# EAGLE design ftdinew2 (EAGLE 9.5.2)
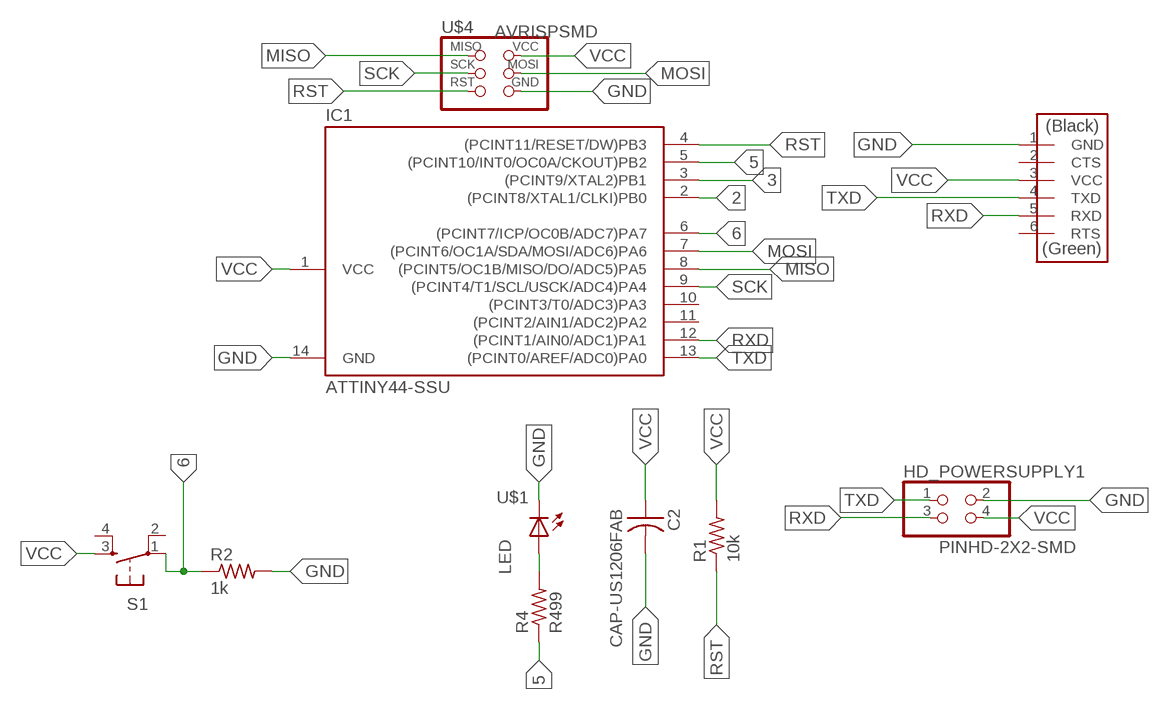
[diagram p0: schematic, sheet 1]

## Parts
C2  CAP-US1206FAB  [C1206FAB]
HD_POWERSUPPLY1  PINHD-2X2-SMD  [2X02SMD]
IC1  ATTINY44-SSU  [SOIC14]
R1  10k  RES-US1206  [R1206]
R2  1k  RES-US1206  [R1206]
R4  R499  RES-US1206  [R1206]
S1  6MM_SWITCH6MM_SWITCH  [6MM_SWITCH]
U$1  LED  [LED1206]
U$4  AVRISPSMD  [2X03SMD]
U$5  FTDI-SMD-HEADER  [1X06SMD]

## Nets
2: IC1.2((PCINT8/XTAL1/CLKI)PB0)
3: IC1.3((PCINT9/XTAL2)PB1)
5: IC1.5((PCINT10/INT0/OC0A/CKOUT)PB2) R4.1
6: IC1.6((PCINT7/ICP/OC0B/ADC7)PA7) R2.1 S1.1(P)
GND: C2.2 HD_POWERSUPPLY1.2 IC1.14(GND) R2.2 U$1.2(C) U$4.6(GND) U$5.1(GND)
MISO: IC1.8((PCINT5/OC1B/MISO/DO/ADC5)PA5) U$4.1(MISO)
MOSI: IC1.7((PCINT6/OC1A/SDA/MOSI/ADC6)PA6) U$4.4(MOSI)
N$1: R4.2 U$1.1(A)
RST: IC1.4((PCINT11/RESET/DW)PB3) R1.1 U$4.5(RST)
RXD: HD_POWERSUPPLY1.3 IC1.12((PCINT1/AIN0/ADC1)PA1) U$5.5(RXD)
SCK: IC1.9((PCINT4/T1/SCL/USCK/ADC4)PA4) U$4.3(SCK)
TXD: HD_POWERSUPPLY1.1 IC1.13((PCINT0/AREF/ADC0)PA0) U$5.4(TXD)
VCC: C2.1 HD_POWERSUPPLY1.4 IC1.1(VCC) R1.2 S1.3(S) U$4.2(VCC) U$5.3(VCC)
Unconnected: IC1.10((PCINT3/T0/ADC3)PA3) IC1.11((PCINT2/AIN1/ADC2)PA2) S1.2(P1) S1.4(S1) U$5.2(CTS) U$5.6(RTS)

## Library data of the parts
C2 = fab:CAP-US
HD_POWERSUPPLY1 = fab:PINHD-2X2-SMD
IC1 = files_fab:ATTINY44
R1 R2 R4 = files_fab:RES-US: Resistor (US Symbol)
S1 = fab:6MM_SWITCH: OMRON SWITCH
U$1 = files_fab:LED: LED
U$4 = files_fab:AVRISP
U$5 = files_fab:FTDI-SMD-HEADER

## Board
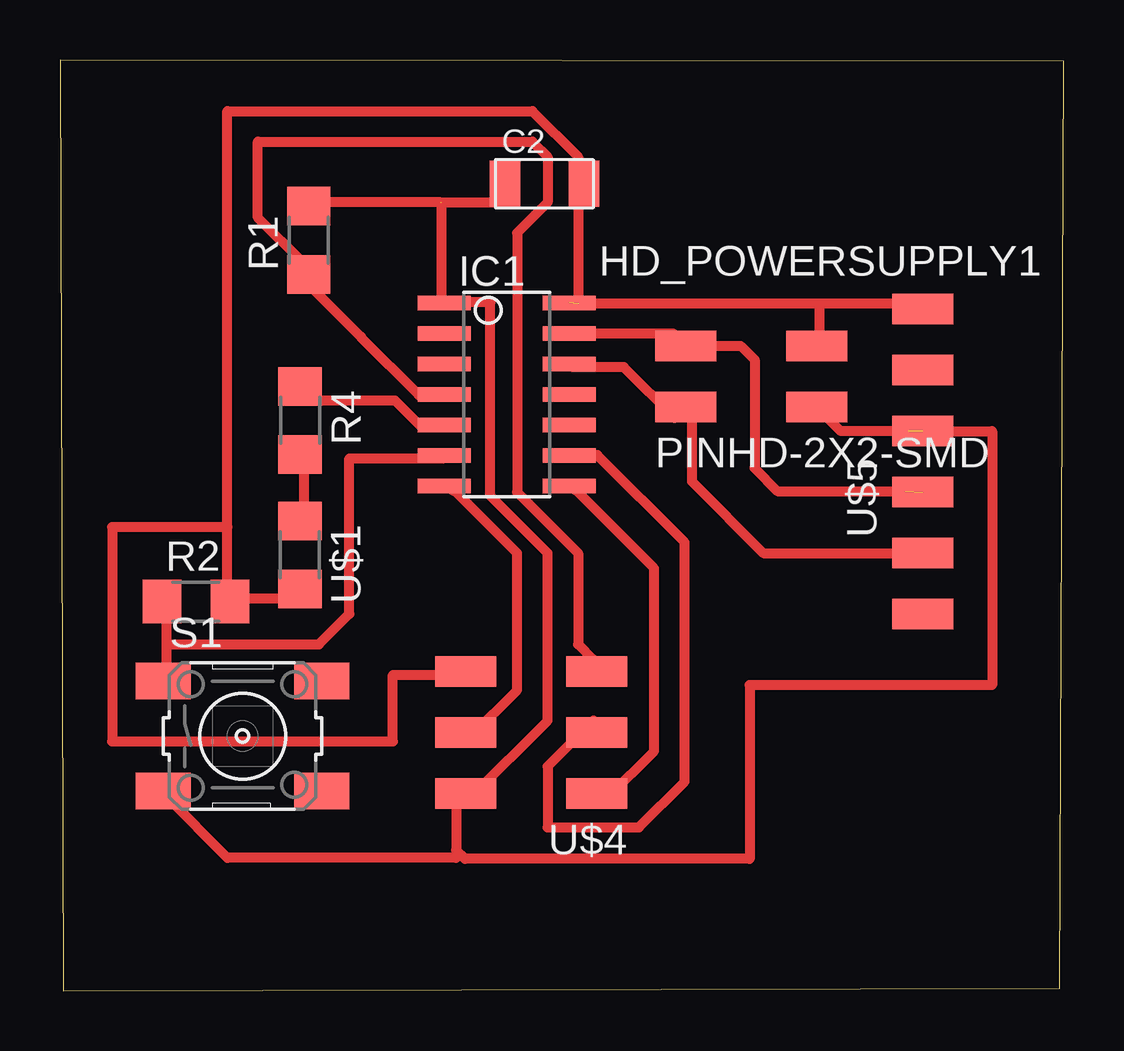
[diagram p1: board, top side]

Size 41.83 x 38.78 mm. Coordinates in mm from the lower left corner, seen from the top.
Outline: 0.13,0 41.65,0.11 41.83,38.72 0,38.78 0.13,0
Copper layers (1*16): Top 0.035mm / dielectric 1.5mm / Bottom 0.035mm
Design rules "default *": minimum track width 16mil, minimum drill 0.35mm, track to track 16mil, track to pad 16mil, pad to pad 16mil, via to via 16mil, smd to smd 16mil, copper to edge 16mil, drill to drill 6mil, minimum pad ring 10mil, minimum via ring 8mil, stop-mask expansion 4mil, vias tented up to drill 0mil, thermal gap 10mil

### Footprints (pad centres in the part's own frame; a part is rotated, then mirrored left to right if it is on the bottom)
C1206FAB = smd 1.27 x 1.905: 1 -1.651,0; 2 1.651,0
2X02SMD = smd 2.54 x 1.27: 1 -2.54,1.27; 2 2.92,1.27; 3 -2.54,-1.27; 4 2.92,-1.27
SOIC14 = smd 0.61 x 2.21: 1 -3.81,-2.603; 2 -2.54,-2.603; 3 -1.27,-2.603; 4 0,-2.603; 5 1.27,-2.603; 6 2.54,-2.603; 7 3.81,-2.603; 8 3.81,2.603; 9 2.54,2.603; 10 1.27,2.603; 11 0,2.603; 12 -1.27,2.603; 13 -2.54,2.603; 14 -3.81,2.603
R1206 = smd 1.6 x 1.803: 1 -1.422,0; 2 1.422,0
6MM_SWITCH = smd 2.286 x 1.524: 1 -3.302,2.286; 2 3.302,2.286; 3 -3.302,-2.286; 4 3.302,-2.286
LED1206 = smd 1.6 x 1.803: 1 -1.422,0; 2 1.422,0
2X03SMD = smd 2.54 x 1.27: 1 -2.54,2.54; 2 2.92,2.54; 3 -2.54,0; 4 2.92,0; 5 -2.54,-2.54; 6 2.92,-2.54
1X06SMD = smd 2.54 x 1.27: 1 0,6.35; 2 0,3.81; 3 0,1.27; 4 0,-1.27; 5 0,-3.81; 6 0,-6.35

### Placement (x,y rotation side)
C2  20.18,33.62 0 top
HD_POWERSUPPLY1  28.6,25.6 0 top
IC1  18.62,24.85 270 top
R1  10.36,31.27 90 top
R2  5.67,16.22 0 top
R4  10,23.76 270 top
S1  7.61,10.61 0 top
U$1  10,18.16 270 top
U$4  19.83,10.75 180 top
U$5  35.94,22.05 0 top

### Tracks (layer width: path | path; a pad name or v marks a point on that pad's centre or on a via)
5
  Top 0.406: R4.1 10.15,24.59 13.96,24.59 15.03,23.52 15.98,23.52 IC1.5
6
  Top 0.406: 4.44,14.43 4.44,13.16 S1.1 | 4.44,14.43 4.44,15.7 R2.1 | 4.44,14.43 10.79,14.43 12.06,15.7 12.06,22.19 15.95,22.19 IC1.6
GND  (2 unrouted)
  Top 0.406: 21.61,28.62 21.61,33.49 C2.2 21.58,34.11 21.58,34.75 19.68,36.65 6.98,36.65 6.98,19.32 | U$5.1 35.72,28.62 31.65,28.62 | 31.65,28.62 21.58,28.62 | U$1.2 9.52,16.33 7.61,16.33 R2.2 6.98,16.33 6.98,19.32 | 6.98,19.32 2.17,19.32 2.17,10.39 13.87,10.39 13.87,13.16 16.5,13.16 U$4.6 | HD_POWERSUPPLY1.2 31.65,26.99 31.65,28.62
MISO
  Top 0.406: IC1.8 21.58,20.78 24.76,17.6 24.76,9.98 22.85,8.08 U$4.1
MOSI
  Top 0.406: IC1.7 16.5,20.78 19.04,18.24 19.04,12.52 17.14,10.62 U$4.4
N$1
  Top 0.406: U$1.1 10.15,20.14 10.15,22.05 R4.2
RST
  Top 0.406: IC1.4 16.01,24.82 14.94,24.82 12.53,27.23 12.53,27.25 10.36,29.43 R1.1 10.15,30.3 8.25,32.21 8.25,35.38 19.68,35.38 20.31,34.75 20.31,32.84 19.04,31.57 19.04,20.78 21.58,18.24 21.58,14.43 22.22,13.79 U$4.5
RXD
  Top 0.406: IC1.12 21.36,25.99 23.5,25.99 25.61,23.87 HD_POWERSUPPLY1.3 26.33,24.07 26.33,21.22 29.3,18.24 U$5.5
SCK
  Top 0.406: IC1.9 21.24,22.32 22.39,22.32 26.03,18.68 26.03,8.71 24.12,6.81 20.31,6.81 20.31,9.35 22.22,11.25 U$4.3
TXD  (1 unrouted)
  Top 0.406: 21.25,27.42 IC1.13 25.55,27.39 HD_POWERSUPPLY1.1 28.36,26.87 28.94,26.29 28.94,21.77 29.89,20.82 35.22,20.82
VCC  (2 unrouted)
  Top 0.406: 15.87,32.84 10.79,32.84 R1.2 | C2.1 18.41,33.48 18.41,32.84 15.89,32.84 15.89,28.66 IC1.1 16.04,28.68 17.93,28.68 17.93,20.62 20.31,18.24 20.31,11.25 17.14,8.08 U$4.2 16.5,8.08 16.5,5.86 | 16.5,5.86 16.5,5.54 6.98,5.54 4.44,8.08 S1.3 | U$5.3 38.84,23.32 38.84,12.73 28.73,12.73 28.73,5.49 16.88,5.49 16.5,5.86 | 35.36,23.32 32.53,23.32 HD_POWERSUPPLY1.4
